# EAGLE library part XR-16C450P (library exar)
UART
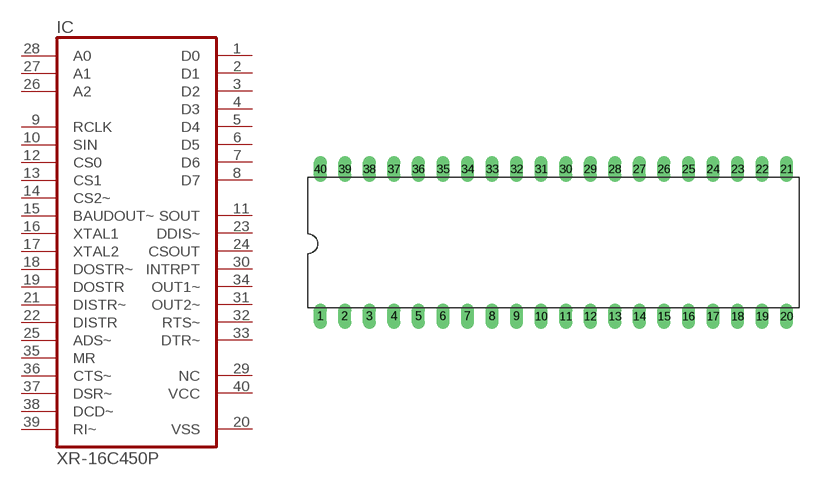
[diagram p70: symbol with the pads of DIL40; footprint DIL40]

Designator prefix IC

## XR-16C450P (MPN: ST16C450CP40; OC_FARNELL: 1209618; OC_NEWARK: 24R1445)  [DIL40]
1  D0
2  D1
3  D2
4  D3
5  D4
6  D5
7  D6
8  D7
9  RCLK  in
10  SIN  in
11  SOUT  out
12  CS0  in
13  CS1  in
14  CS2~  in
15  BAUDOUT~  in
16  XTAL1  in
17  XTAL2  in
18  DOSTR~  in
19  DOSTR  in
20  VSS  pwr
21  DISTR~  in
22  DISTR  in
23  DDIS~  out
24  CSOUT  out
25  ADS~  in
26  A2  in
27  A1  in
28  A0  in
29  NC  nc
30  INTRPT  out
31  OUT2~  out
32  RTS~  out
33  DTR~  out
34  OUT1~  out
35  MR  in
36  CTS~  in
37  DSR~  in
38  DCD~  in
39  RI~  in
40  VCC  pwr

## Footprint DIL40 (pad centres in mm)
Dual In Line Package
drill 0.813 long: 1 -24.13,-7.62; 2 -21.59,-7.62; 3 -19.05,-7.62; 4 -16.51,-7.62; 5 -13.97,-7.62; 6 -11.43,-7.62; 7 -8.89,-7.62; 8 -6.35,-7.62; 9 -3.81,-7.62; 10 -1.27,-7.62; 11 1.27,-7.62; 12 3.81,-7.62; 13 6.35,-7.62; 14 8.89,-7.62; 15 11.43,-7.62; 16 13.97,-7.62; 17 16.51,-7.62; 18 19.05,-7.62; 19 21.59,-7.62; 20 24.13,-7.62; 21 24.13,7.62; 22 21.59,7.62; 23 19.05,7.62; 24 16.51,7.62; 25 13.97,7.62; 26 11.43,7.62; 27 8.89,7.62; 28 6.35,7.62; 29 3.81,7.62; 30 1.27,7.62; 31 -1.27,7.62; 32 -3.81,7.62; 33 -6.35,7.62; 34 -8.89,7.62; 35 -11.43,7.62; 36 -13.97,7.62; 37 -16.51,7.62; 38 -19.05,7.62; 39 -21.59,7.62; 40 -24.13,7.62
